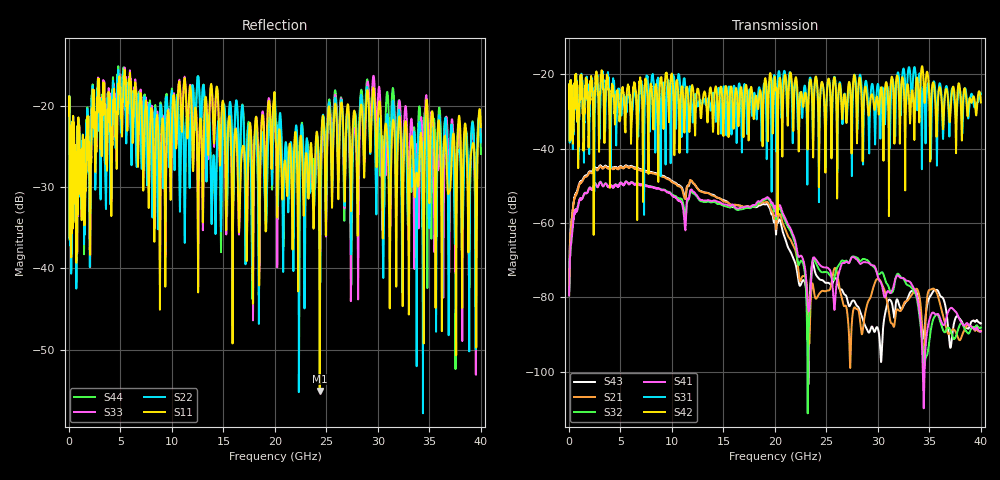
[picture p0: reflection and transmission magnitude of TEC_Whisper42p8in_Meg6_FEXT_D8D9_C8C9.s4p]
! Tyco Electronics Strada Whisper System
! FEXT_D8D9-C8C9
!! SYSTEM DESCRIPTION: Daughtercard-Connector-Backplane-Connector-Daughtercard
!! PCB DESCRIPTION: BP: 250mil, 26 lyrs, Megtron6, bottom layer route, no stub, 6-9-6mil 30" traces; DC: 150mil, 16 lyrs, Megtron6, bottom layer route, no stub, 6-9-6mil 5" traces
!! CONNECTOR DESCRIPTION: STRADA Whisper, Right Angle Receptacle to Vertical Header
!! MODEL DESCRIPTION: Tyco Electronics System 4-port S-parameter
!! MODEL STATUS: Developmental
!! MODEL GEOMETRY: Channel Model
!! MODEL FREQUENCY RANGE: DC to 40 GHz in 10 MHz frequency steps
!! MODEL EDGE RATE LIMITATION: 12.5 ps (Using conservative 0.5/Fmax rule of thumb)
!! TIME-DOMAIN TRANSFORM CAUTIONS:
!! 1.) Do not simulate transient edge rates faster than the number listed above.  Edge rates faster than this number
!!  contain significant spectral content at frequencies above the model's highest frequency.
!! 2.) Even when simulating edge rates that are slower than the number listed above, be aware that the best time
!!  resolution possible with a direct iFFT is (1 / 2Fmax).  As a result, time resolution is typically not adequate
!!  for most time-domain simulations unless tricks such as windowing are used to minimize leakage and aliasing.
!! 3.) Because the model has a uniform frequency step, a direct iFFT will result in an impulse that that has a time
!!  length given by either (1 / Fstep) or (1 / 2Fstep), depending on the transform being used.  Care has been taken
!!  in selecting the frequency step to ensure a settled impulse response for the model.  Therefore, convolution with
!!  the model's impulse response should present no issues.  However, if directly concatenating s-parameter models
!!  in the frequency domain a user must either interpolate necessary interim frequencies or complete impulse response
!!  zero-padding.  Impulse response zero-padding is more difficult, but more accurate.
!! PORT DEFINITIONS:
!! Port  1  ----->  Side A  C8  D8  Side B  <-----  Port  2
!! Port  3  ----->  Side A  C9  D9  Side B  <-----  Port  4
! Created Wed Apr 27 14:00:04 2011
# hz S ma R 50
! 4 Port Network Data from SP1.SP block
! freq  magS11  angS11  magS12  angS12  magS13  angS13  magS14  angS14
!  magS21  angS21  magS22  angS22  magS23  angS23  magS24  angS24
!  magS31  angS31  magS32  angS32  magS33  angS33  magS34  angS34
!  magS41  angS41  magS42  angS42  magS43  angS43  magS44  angS44
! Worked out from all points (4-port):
!   4000 points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, 10 MHz to 40 GHz, reference 50 ohm
!   strongest paths, dB at 10 MHz, 10.01 GHz, 20.01 GHz, 30.01 GHz, 40 GHz:
!     S42: -29.2, -20.2, -21.2, -28.2, -27.6
!     S31: -29.3, -22.6, -23.1, -22.6, -25.3
!     S41: -79.5, -52.7, -55.3, -74.6, -89.2
!     S32: -79.4, -52.4, -56.3, -73.7, -88.2
!     S21: -78.4, -49.1, -57.9, -75.2, -89.0
!     S43: -78.3, -48.8, -59.5, -88.6, -87.0
!   lowest |S11| = -55.1 dB at 24.35 GHz (marker M1), VSWR 1.00, Z = 50 + j0.175 ohm
!   |S11| at or under -10 dB: start of sweep to end of sweep
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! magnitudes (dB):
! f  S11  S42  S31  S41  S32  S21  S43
! 10 MHz  -21.2  -29.2  -29.3  -79.5  -79.4  -78.4  -78.3
! 1.11 GHz  -30.2  -20.5  -21.1  -53.5  -53.4  -49.2  -48.9
! 6.04 GHz  -18.4  -36.4  -31.0  -49.0  -49.0  -44.8  -44.6
! 19.27 GHz  -21.7  -33.1  -29.6  -53.1  -53.4  -54.3  -55.0
! 23.26 GHz  -31.4  -27.0  -25.1  -83.7  -89.7  -86.3  -97.6
! 24.35 GHz  -55.1  -29.3  -29.5  -71.3  -72.8  -78.9  -75.2
! 40 GHz  -22.6  -27.6  -25.3  -89.2  -88.2  -89.0  -87.0
